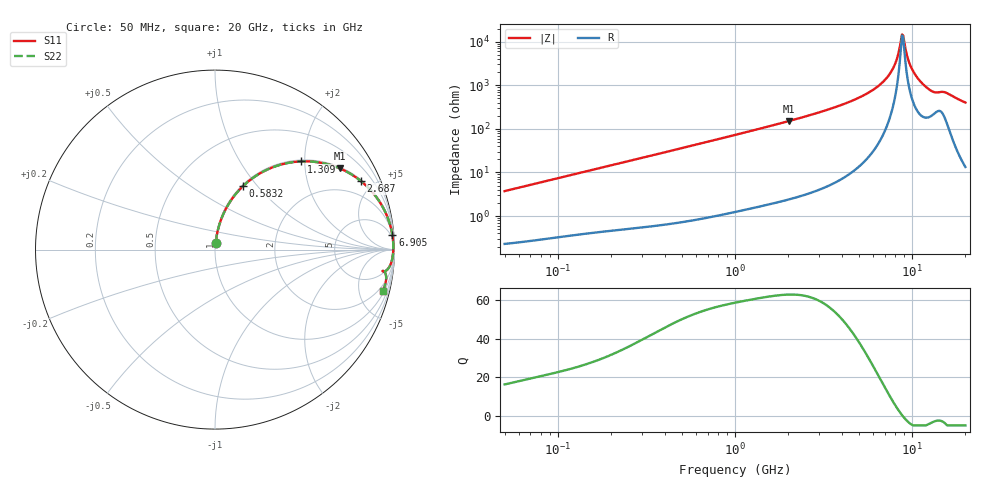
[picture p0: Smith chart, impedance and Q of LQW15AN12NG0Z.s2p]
!Murata Part Number: LQW15AN12NG0Z
!These Parameters are Measured in Series Mode Connection
!  o--[Z]--o
!Port1  Port2
!  o-------o
!Freq. Start=50[MHz] Stop=20[GHz], 401[Steps]
# Hz S RI R 50
!Freq.(Hz) S11(Real) S11(Imag) S21(Real) S21(Imag) S12(Real) S12(Imag) S22(Real) S22(Imag)
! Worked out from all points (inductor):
!   401 points, 50 MHz to 20 GHz, reference 50 ohm
!   read as one part in series: L = 11.8 nH near 51.52 MHz
!   highest Q = 62.8 at 2.022 GHz (marker M1), where L = 12 nH
!   self-resonance near 8.775 GHz
!   S11 on the Smith chart (normalised r, x): 50 MHz: 1.00, +0.07; 583.2 MHz: 1.02, +0.84; 1.309 GHz: 1.03, +1.91; 2.687 GHz: 1.07, +4.20; 6.905 GHz: 3, +25; 20 GHz: 1.27, -8.04
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5e7  0.00368 0.0371  0.9963 -0.0371  0.9963 -0.0371  0.00368 0.0371
1.364002e8  0.0136 0.0982  0.9864 -0.0982  0.9864 -0.0982  0.0136 0.0982
3.721004e8  0.0725 0.2482  0.9275 -0.2482  0.9275 -0.2482  0.0725 0.2482
5.831961e8  0.1557 0.3531  0.8443 -0.3531  0.8443 -0.3531  0.1557 0.3531
1e9  0.3476 0.4677  0.6524 -0.4677  0.6524 -0.4677  0.3476 0.4677
1.309461e9  0.4784 0.4914  0.5216 -0.4914  0.5216 -0.4914  0.4784 0.4914
2.021818e9  0.6947 0.4526  0.3053 -0.4526  0.3053 -0.4526  0.6947 0.4526
2.687447e9  0.8116 0.383  0.1884 -0.383  0.1884 -0.383  0.8116 0.383
2.728004e9  0.8169 0.3787  0.1831 -0.3787  0.1831 -0.3787  0.8169 0.3787
4.89267e9  0.9566 0.1915  0.0434 -0.1915  0.0434 -0.1915  0.9566 0.1915
5.944466e9  0.9784 0.1279  0.0216 -0.1279  0.0216 -0.1279  0.9784 0.1279
6.905011e9  0.9885 0.0796  0.0115 -0.0796  0.0115 -0.0796  0.9885 0.0796
7.442007e9  0.9916 0.0555  0.00839 -0.0555  0.00839 -0.0555  0.9916 0.0555
8.141811e9  0.9935 0.0265  0.00647 -0.0265  0.00647 -0.0265  0.9935 0.0265
8.644534e9  0.9937 0.007  0.00633 -0.007  0.00633 -0.007  0.9937 0.007
8.907419e9  0.9934 -0.00279  0.00662 0.00279  0.00662 0.00279  0.9934 -0.00279
9.457416e9  0.992 -0.0225  0.00805 0.0225  0.00805 0.0225  0.992 -0.0225
9.892087e9  0.9901 -0.0375  0.00995 0.0375  0.00995 0.0375  0.9901 -0.0375
1.149051e10  0.9758 -0.088  0.0242 0.088  0.0242 0.088  0.9758 -0.088
1.295331e10  0.9481 -0.1201  0.0519 0.1201  0.0519 0.1201  0.9481 -0.1201
1.527346e10  0.9467 -0.1269  0.0533 0.1269  0.0533 0.1269  0.9467 -0.1269
2e10  0.935 -0.2305  0.065 0.2305  0.065 0.2305  0.935 -0.2305
